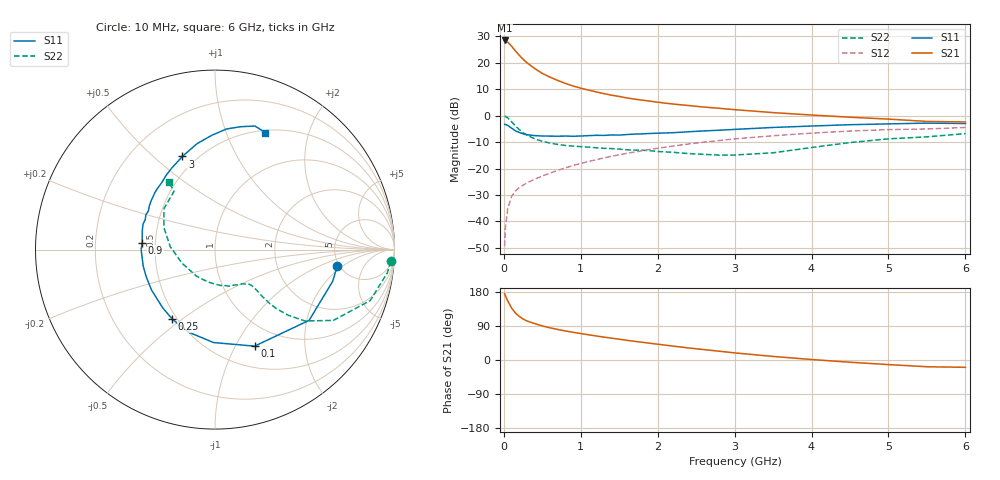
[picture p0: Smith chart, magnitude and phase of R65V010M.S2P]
! SIEMENS Small Signal Semiconductors
! BFR193
! Si NPN RF Bipolar Junction Transistor in SOT23
! VCE = 5 V  IC = 10 mA
! Common Emitter S-Parameters:  May  1996
# GHz  S  MA  R  50
!  f  S11  S21  S12  S22
! GHz  MAG  ANG  MAG  ANG  MAG  ANG  MAG  ANG
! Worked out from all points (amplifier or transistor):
!   36 points, 10 MHz to 6 GHz, reference 50 ohm
!   highest |S21| = 28.5 dB at 10 MHz (marker M1)
!   |S21| within 3 dB of that: start of sweep to 123.7 MHz
!   unconditionally stable (mu >= 1): 736.7 MHz to 2.007 GHz
!   at 250 MHz: K = 0.64, MSG = 23.8 dB, |S12| = -26.3 dB
!   at 1.4 GHz: K = 1.04, MAG = 10.4 dB, |S12| = -15.4 dB
!   at 6 GHz: K = 0.94, MSG = 1.0 dB, |S12| = -4.5 dB
!   lowest NFmin = 1.30 dB at 450 MHz
!   S11 on the Smith chart (normalised r, x): 10 MHz: 4.79, -1.67; 100 MHz: 0.74, -1.20; 250 MHz: 0.47, -0.46; 900 MHz: 0.42, +0.04; 3 GHz: 0.42, +0.62; 6 GHz: 0.53, +1.38
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0.01  0.6875 -7.7  26.47 174.9  0.0034 83.0  0.9818 -3.8
0.02  0.6789 -15.1  26.24 169.7  0.0075 80.8  0.9684 -7.7
0.05  0.6561 -36.9  24.63 156.1  0.0171 72.9  0.9099 -18.2
0.1  0.5814 -67.7  20.68 137.5  0.0296 63.4  0.7683 -30.9
0.15  0.5179 -90.9  16.8 124.0  0.0376 58.5  0.6399 -38.4
0.2  0.4828 -107.9  13.91 115.1  0.0435 56.5  0.5477 -41.9
0.25  0.4545 -121.6  11.68 108.2  0.0484 55.5  0.4772 -43.8
0.3  0.4361 -131.9  10.04 103.1  0.0533 56.6  0.4272 -44.6
0.4  0.4193 -147.4  7.799 96.1  0.063 57.9  0.3653 -44.7
0.5  0.4124 -157.7  6.309 90.0  0.072 59.4  0.3273 -44.3
0.6  0.4105 -167.0  5.349 84.9  0.0821 60.9  0.303 -44.2
0.7  0.4084 -174.3  4.642 80.6  0.0921 62.2  0.2861 -44.5
0.9  0.4079 174.5  3.646 73.1  0.1143 62.6  0.2654 -45.8
1.1  0.4191 165.0  3.048 66.6  0.136 63.0  0.2539 -49.0
1.3  0.4232 156.6  2.613 60.5  0.1589 62.2  0.2415 -52.6
1.6  0.4395 146.3  2.165 51.9  0.1939 60.4  0.2267 -60.3
2.2  0.4763 128.7  1.658 36.7  0.2666 54.7  0.2027 -80.7
3  0.5501 109.3  1.3 18.8  0.3638 44.1  0.1802 -124.4
3.5  0.5982 99.7  1.142 9.4  0.4173 36.6  0.1984 -157.2
4.5  0.6749 84.6  0.935 -5.9  0.5121 21.8  0.3099 156.7
5.5  0.7235 72.1  0.778 -17.8  0.5598 6.3  0.3973 125.0
6  0.71 66.7  0.761 -19.3  0.5982 1.7  0.4582 124.3
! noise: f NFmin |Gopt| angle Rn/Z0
0.45  1.3  0.22  143  0.11
0.9  1.3  0.34  160  0.11
1.8  2.05  0.54  -153  0.14
